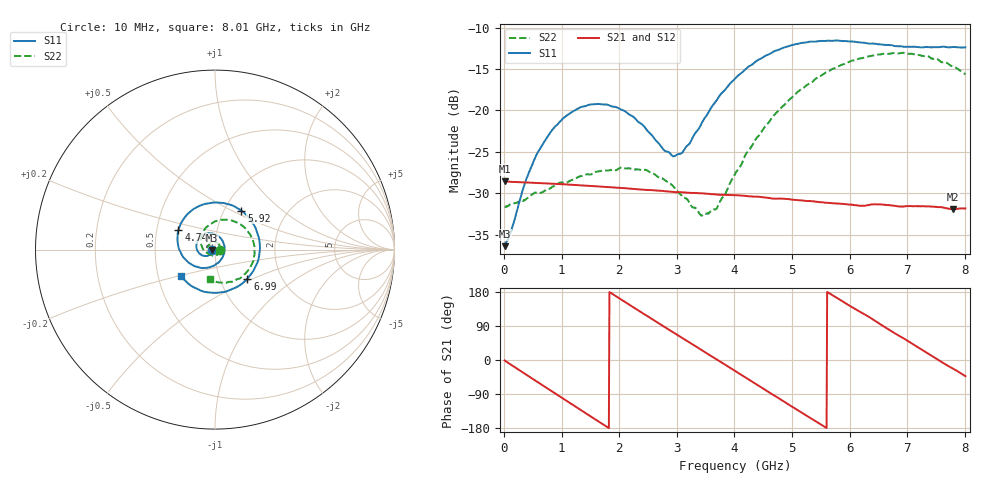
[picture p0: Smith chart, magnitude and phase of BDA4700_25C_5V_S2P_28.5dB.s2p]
!Agilent Technologies,E5071B,MY42404982,A.09.10
!Date: Mon Oct 20 13:40:55 2025
!Data & Calibration Information:
!Freq	S11:SOLT2(ON)	S21:SOLT2(ON)	S12:SOLT2(ON)	S22:SOLT2(ON)
# Hz S RI R 50
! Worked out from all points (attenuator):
!   801 points, 10 MHz to 8.01 GHz, reference 50 ohm
!   highest |S21| = -28.56 dB at 10 MHz (marker M1); lowest = -31.9 dB at 7.8 GHz (marker M2)
!   lowest |S11| = -36.4 dB at 10 MHz (marker M3), VSWR 1.03, Z = 48.5 - j0.128 ohm
!   |S11| at or under -10 dB: start of sweep to end of sweep
!   |S22| runs from -32.7 to -13.0 dB; largest |S21 - S12| = 0.00031
!   S11 on the Smith chart (normalised r, x): 10 MHz: 0.97, -0.00; 4.74 GHz: 0.65, +0.15; 5.92 GHz: 1.20, +0.56; 6.99 GHz: 1.35, -0.46; 8.01 GHz: 0.65, -0.20
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1e7  -0.0151 -0.00132  0.0373 -0.0008  0.0373 -0.000842  0.0262 -0.000797
1.3e8  -0.0164 -0.00988  0.036 -0.00854  0.036 -0.00856  0.0266 -0.00625
3.8e8  -0.0268 -0.0268  0.0289 -0.0227  0.0288 -0.0227  0.0214 -0.0197
5.9e8  -0.0433 -0.0357  0.0188 -0.0312  0.0188 -0.0312  0.0134 -0.029
1e9  -0.0845 -0.0235  -0.00585 -0.0354  -0.0059 -0.0354  -0.0146 -0.0338
1.35e9  -0.1042 0.0144  -0.0244 -0.0254  -0.0245 -0.0255  -0.036 -0.0178
2.07e9  -0.0426 0.0905  -0.031 0.0138  -0.0311 0.0138  -0.0305 0.0331
2.68e9  0.0433 0.0464  -0.00426 0.0325  -0.00429 0.0325  0.0127 0.0374
2.93e9  0.0529 0.00201  0.00907 0.0309  0.00908 0.0309  0.0247 0.0248
3.06e9  0.0498 -0.0229  0.0154 0.0281  0.0153 0.0282  0.0274 0.0149
3.44e9  0.00133 -0.0849  0.0286 0.0135  0.0286 0.0135  0.0187 -0.0139
3.69e9  -0.0532 -0.1018  0.0311 0.000842  0.0311 0.000763  0.000638 -0.0255
4.01e9  -0.1314 -0.0826  0.027 -0.0148  0.027 -0.0148  -0.0321 -0.0257
4.74e9  -0.2036 0.1085  -0.00422 -0.0291  -0.00413 -0.0291  -0.0793 0.0571
5.35e9  -0.0602 0.2531  -0.0259 -0.0115  -0.0259 -0.0115  -0.0154 0.1476
5.92e9  0.1466 0.2176  -0.0237 0.0133  -0.0238 0.0133  0.1116 0.1557
6.28e9  0.2307 0.1083  -0.0129 0.0233  -0.0126 0.0234  0.1844 0.0997
6.68e9  0.2426 -0.0517  0.00452 0.0264  0.00457 0.0265  0.2198 0.00013
6.99e9  0.1803 -0.1613  0.0162 0.0209  0.0163 0.0208  0.2045 -0.0825
7.39e9  0.0366 -0.2381  0.0255 0.00659  0.0255 0.00657  0.1323 -0.1625
7.8e9  -0.1297 -0.2035  0.0232 -0.0101  0.0233 -0.0101  0.0207 -0.1826
8.01e9  -0.1917 -0.1449  0.0188 -0.0174  0.0188 -0.0173  -0.0299 -0.1621
